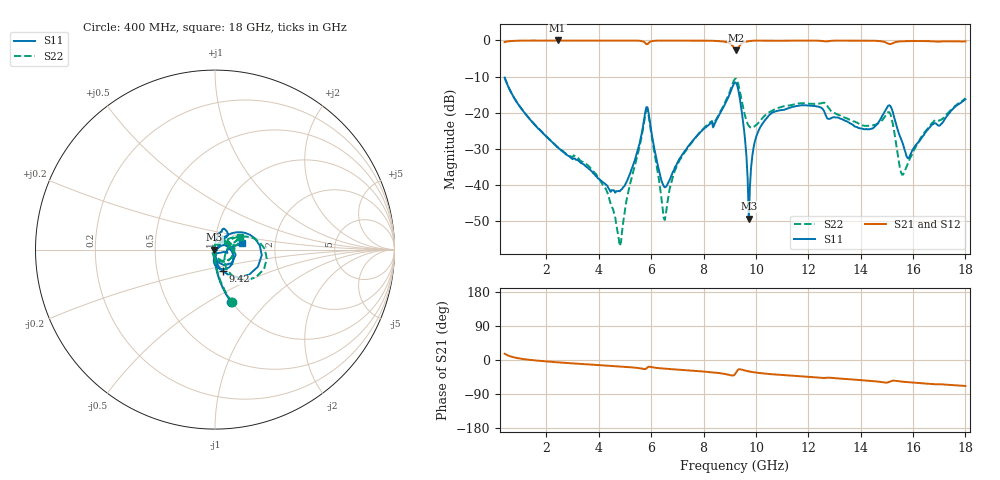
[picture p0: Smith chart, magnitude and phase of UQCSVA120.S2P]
!  Part Number  UQCSVA120  Mounting Orientation: Horizontal
!  Description: Ultra Low ESR Microwave capacitors
!  Application: Coupling, Bypass, Tuning, DC Block
!  Filters, Matching
# GHZ S DB R 50
! Freq  |S11|  S11 Ph  |S21|  S21 Ph  |S12|  S12 Ph  |S22|  S22 Ph
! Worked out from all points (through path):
!   401 points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, 400 MHz to 18 GHz, reference 50 ohm
!   highest |S21| = -0.04 dB at 2.424 GHz (marker M1); lowest = -2.8 dB at 9.244 GHz (marker M2)
!   group delay of S21, straight-line fit = 11.3 ps
!   lowest |S11| = -49.2 dB at 9.728 GHz (marker M3), VSWR 1.01, Z = 49.7 - j0.0221 ohm
!   |S11| at or under -10 dB: start of sweep to end of sweep
!   |S22| runs from -56.9 to -10.3 dB; largest |S21 - S12| = 0.005
!   S11 on the Smith chart (normalised r, x): 400 MHz: 0.99, -0.64; 9.42 GHz: 1.06, -0.26; 18 GHz: 1.34, +0.10
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0.4  -10.30 -72.7  -0.48 16.7  -0.48 16.7  -10.27 -71.9
2.424  -29.57 -88.0  -0.04 -6.2  -0.05 -6.2  -29.48 -93.3
3.348  -33.97 -90.2  -0.05 -10.5  -0.05 -10.5  -33.50 -92.2
4.272  -39.89 -68.9  -0.05 -14.7  -0.04 -14.7  -41.09 -104.7
4.8  -41.71 -22.3  -0.05 -17.1  -0.04 -17.1  -56.87 167.4
5.812  -18.49 -14.5  -1.02 -22.6  -1.00 -22.6  -19.22 5.0
6.296  -35.94 -73.0  -0.08 -21.6  -0.08 -21.6  -38.53 -81.0
6.516  -40.61 -24.0  -0.07 -22.9  -0.06 -22.9  -49.64 -6.2
7.088  -32.57 40.0  -0.06 -25.8  -0.06 -25.8  -33.09 57.3
9.2  -11.62 -6.8  -2.53 -37.6  -2.51 -37.6  -10.67 -9.9
9.244  -11.78 -21.6  -2.77 -32.9  -2.73 -32.8  -10.63 -21.7
9.42  -17.78 -69.8  -1.12 -24.7  -1.11 -24.8  -15.32 -56.6
9.728  -49.24 -176.3  -0.23 -30.1  -0.23 -30.1  -23.66 -33.3
9.992  -27.09 84.5  -0.09 -33.1  -0.08 -33.1  -23.45 0.1
10.432  -21.26 77.7  -0.09 -36.5  -0.09 -36.6  -20.28 18.1
12.148  -18.08 62.2  -0.09 -45.1  -0.07 -45.1  -17.56 23.2
14.216  -24.51 36.4  -0.11 -54.0  -0.10 -54.1  -23.64 29.9
15.096  -17.94 -51.3  -1.04 -57.8  -1.02 -57.8  -19.87 -26.7
15.624  -28.84 -91.9  -0.26 -57.4  -0.24 -57.4  -37.08 155.4
15.844  -32.52 -55.7  -0.22 -58.6  -0.21 -58.6  -33.27 100.1
16.636  -24.03 -12.5  -0.24 -63.0  -0.23 -63.0  -23.71 56.0
18  -16.31 14.3  -0.31 -68.5  -0.31 -68.5  -16.05 27.5
